FUNCTION_BLOCK FB82
TITLE =Get Velocity Profile
//*****************************************************************************
//* maxon motor ag
//* R&D
//* all rights reserved
//*****************************************************************************
//* Summary:  Get Velocity Profile
//*
//* Remarks:
//*
//* Created under: STEP7 REV5.2+SP1
//*****************************************************************************
//* History:
//* 19.05.2004 | INA   first release
//*
//*
//*****************************************************************************
//

AUTHOR:INA
FAMILY:ProVeloM
NAME:GetVeloP
VERSION:00.01


VAR_INPUT

Read : BOOL //A rising edge start the command

  NodeID : BYTE //Adress of the maxon device

END_VAR
VAR_OUTPUT
  Done : BOOL //Data valid flag is TRUE if data were available

  Err : BOOL //Error flag is TRUE if an Error has occured, see ErrNo for more details

  ErrNo : DINT //Contains detailed error information

  ProfileAcceleration : DWORD
  ProfileDeceleration : DWORD
END_VAR
VAR
  xEdgeMerker : BOOL //Edge Merker

  xEdgeFlag : BOOL //Edge Flag

  xStep : INT
END_VAR

BEGIN

NETWORK
TITLE = Activate the service function
//

// SDO Read "Get Velocity Profile"

       U    #Read
       FP   #xEdgeFlag                   // recognize a positiv edge of the Read signal
       =    #xEdgeMerker                 // and set the xEdgeMerker for one cycle to true

       L    #xStep
       L    0
       ==I
       U    #xEdgeMerker
       SPB  nstp                         // iStep = 1 -> fnc1

       L    #xStep                       // jump list
       SPL  List
       SPA  rdef
       SPA  fnc1
       SPA  fncE
List  :SPA  rdef

rdef  :NOP  0
       R    #Done                        // reset Done
       R    #Err                         // reset Error
       L    0
       T    #xStep                       // iStep = 0
       SPA  end

fnc1  :NOP  0
       CALL FC1
         NodeID:=#NodeID
         Index:=DW#16#00006083
         SubIndex:=DW#16#00000000
         RET_VAL:=#Done
         Err:=#Err
         ErrNo:=#ErrNo

       L    DB219.DBD10
       T    #ProfileAcceleration

       L    1
       U    #Err
       SPB  fncE

       NOP  0
       CALL FC1
         NodeID:=#NodeID
         Index:=DW#16#00006084
         SubIndex:=DW#16#00000000
         RET_VAL:=#Done
         Err:=#Err
         ErrNo:=#ErrNo

       L    DB219.DBD10
       T    #ProfileDeceleration

       L    1
       U    #Err
       SPB  fncE

       SPA  nstp                         // iStep = 2 -> fncE

fncE  :NOP  0
       L    0
       T    #xStep
       SPA  end

nstp  :NOP  0
       L    #xStep
       INC            1
       T    #xStep

end   :NOP  0
END_FUNCTION_BLOCK
